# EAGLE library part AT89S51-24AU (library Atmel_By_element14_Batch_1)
MCU
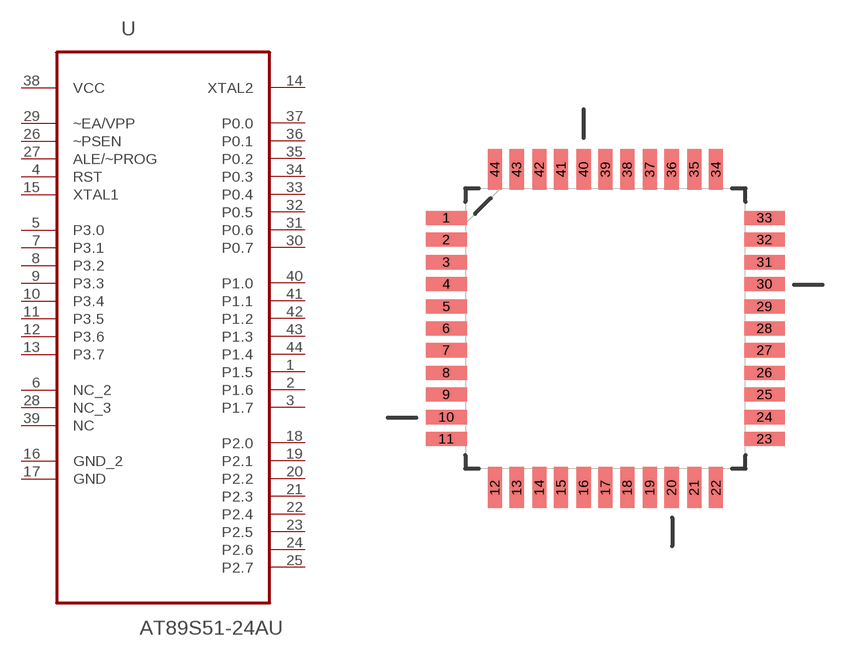
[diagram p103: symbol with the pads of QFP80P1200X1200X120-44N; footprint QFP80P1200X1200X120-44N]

Designator prefix U

## AT89S51-24AU (DESCRIPTION: MCU; MPN: AT89S51-24AU; OC_FARNELL: 1841597; OC_NEWARK: 12T1383; PACKAGE: QFP-44; SUPPLIER: Atmel)  [QFP80P1200X1200X120-44N]
1  P1.5
2  P1.6
3  P1.7
4  RST  in
5  P3.0
6  NC_2  nc
7  P3.1
8  P3.2
9  P3.3
10  P3.4
11  P3.5
12  P3.6
13  P3.7
14  XTAL2  out
15  XTAL1  in
16  GND_2  pas
17  GND  pas
18  P2.0
19  P2.1
20  P2.2
21  P2.3
22  P2.4
23  P2.5
24  P2.6
25  P2.7
26  ~PSEN  in
27  ALE/~PROG  in
28  NC_3  nc
29  ~EA/VPP  in
30  P0.7
31  P0.6
32  P0.5
33  P0.4
34  P0.3
35  P0.2
36  P0.1
37  P0.0
38  VCC  pwr
39  NC  nc
40  P1.0
41  P1.1
42  P1.2
43  P1.3
44  P1.4

## Footprint QFP80P1200X1200X120-44N (pad centres in mm)
smd 1.473 x 0.508: 1 -5.74,3.988; 2 -5.74,3.2; 3 -5.74,2.388; 4 -5.74,1.6; 5 -5.74,0.787; 6 -5.74,0; 7 -5.74,-0.787; 8 -5.74,-1.6; 9 -5.74,-2.388; 10 -5.74,-3.2; 11 -5.74,-3.988; 23 5.74,-3.988; 24 5.74,-3.2; 25 5.74,-2.388; 26 5.74,-1.6; 27 5.74,-0.787; 28 5.74,0; 29 5.74,0.787; 30 5.74,1.6; 31 5.74,2.388; 32 5.74,3.2; 33 5.74,3.988
smd 0.508 x 1.473: 12 -3.988,-5.74; 13 -3.2,-5.74; 14 -2.388,-5.74; 15 -1.6,-5.74; 16 -0.787,-5.74; 17 0,-5.74; 18 0.787,-5.74; 19 1.6,-5.74; 20 2.388,-5.74; 21 3.2,-5.74; 22 3.988,-5.74; 34 3.988,5.74; 35 3.2,5.74; 36 2.388,5.74; 37 1.6,5.74; 38 0.787,5.74; 39 0,5.74; 40 -0.787,5.74; 41 -1.6,5.74; 42 -2.388,5.74; 43 -3.2,5.74; 44 -3.988,5.74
